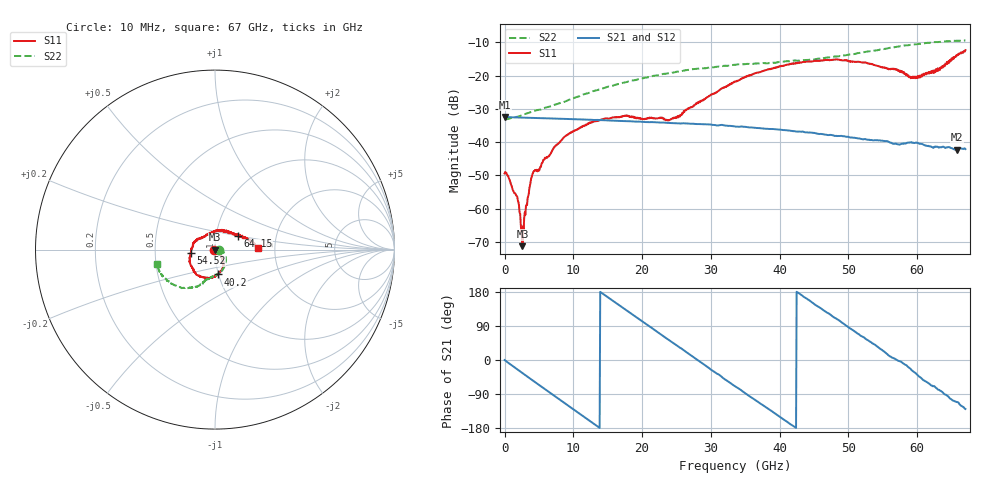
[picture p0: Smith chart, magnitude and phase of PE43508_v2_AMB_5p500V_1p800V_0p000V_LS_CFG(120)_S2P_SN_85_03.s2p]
!Keysight Technologies,N5227A,US51270237,A.10.43.00
!Date: Wednesday, August 22, 2018 17:19:14
!Correction: S11(Full 2 Port(1,3))
!S31(Full 2 Port(1,3))
!S13(Full 2 Port(1,3))
!S33(Full 2 Port(1,3))
!S2P File: Measurements: S11, S31, S13, S33:
# Hz S  dB  R 50
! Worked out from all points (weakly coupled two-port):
!   801 points, 10 MHz to 67 GHz, reference 50 ohm
!   highest |S21| = -32.48 dB at 10 MHz (marker M1); lowest = -42.3 dB at 65.74 GHz (marker M2)
!   lowest |S11| = -71.3 dB at 2.606 GHz (marker M3), VSWR 1.00, Z = 50 - j0.0257 ohm
!   |S11| at or under -10 dB: start of sweep to end of sweep
!   |S22| runs from -33.2 to -9.5 dB; largest |S21 - S12| = 0.00013
!   S11 on the Smith chart (normalised r, x): 10 MHz: 0.99, -0.00; 40.2 GHz: 0.99, -0.28; 54.52 GHz: 0.76, -0.03; 64.15 GHz: 1.27, +0.19; 67 GHz: 1.63, +0.03
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1e7  -49.43 -174.5  -32.48 -0.2  -32.46 -0.2  -33.16 -0.5
1.768488e9  -56.15 163.5  -32.59 -23.7  -32.60 -23.7  -32.42 2.7
2.438388e9  -66.97 -128.6  -32.63 -32.4  -32.64 -32.5  -31.98 1.7
2.605862e9  -71.28 -70.2  -32.65 -34.6  -32.65 -34.7  -31.83 1.9
2.773338e9  -66.44 -46.7  -32.66 -36.8  -32.66 -36.8  -31.70 2.1
3.69445e9  -53.11 -41.4  -32.72 -48.8  -32.72 -48.8  -31.09 0.9
4.196875e9  -48.96 -32.8  -32.74 -55.3  -32.75 -55.3  -30.70 0.5
8.634962e9  -38.60 -62.2  -33.03 -112.5  -33.02 -112.5  -27.92 -8.6
1.123082e10  -35.32 -69.5  -33.20 -145.8  -33.21 -145.8  -25.89 -17.4
1.74274e10  -32.16 -87.6  -33.67 135.0  -33.67 135.0  -22.08 -39.2
2.236791e10  -32.76 -81.3  -34.11 72.0  -34.11 71.9  -19.88 -56.7
2.513125e10  -32.26 -63.9  -34.37 37.3  -34.36 37.2  -18.80 -65.3
3.3505e10  -21.88 -55.9  -35.30 -69.4  -35.30 -69.5  -16.77 -88.5
4.0204e10  -17.13 -83.3  -36.32 -152.1  -36.32 -152.1  -15.86 -100.6
4.472582e10  -15.75 -106.7  -37.19 151.6  -37.15 151.6  -15.23 -105.7
4.841028e10  -15.18 -126.7  -38.18 107.1  -38.17 107.1  -14.27 -109.4
5.452311e10  -17.32 -172.3  -39.47 30.8  -39.44 30.7  -12.22 -120.9
5.586291e10  -18.16 171.5  -39.96 11.8  -39.94 11.3  -11.73 -124.3
5.979858e10  -20.33 113.3  -40.16 -35.1  -40.20 -35.5  -10.63 -136.3
6.415292e10  -16.65 30.4  -41.72 -91.4  -41.78 -91.5  -9.72 -153.0
6.574394e10  -14.09 13.8  -42.28 -111.0  -42.30 -111.6  -9.56 -159.6
6.7e10  -12.37 1.9  -42.10 -129.3  -42.15 -129.3  -9.47 -165.8
